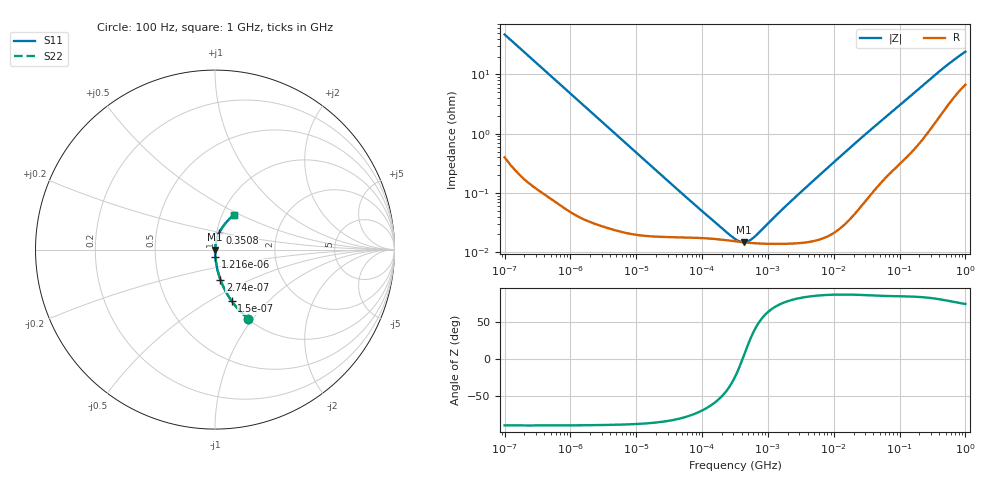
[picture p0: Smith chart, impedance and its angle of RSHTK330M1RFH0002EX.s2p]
! RSHTK330M1RFH0002EX  S-PARAMETER MODEL  (General Type)
! Model Generated by ELNA Corporation (http://www.ty-top.com)
! Version 1.0
! ELNA Control No. 201203
! Copyright (c) 2020 ELNA CO.,LTD. All Rights Reserved.
! Products Name : CONDUCTIVE POLYMER HYBRID ALUMINUM ELECTROLYTIC CAPACITORS
! Characteristics :
!  Capacitance  :  33uF  ,  Rated voltage  :  80V
!  Operating Temp. Range  :  -55 to +125 degC  ,  Endurance  :  4000hr at 125 degC
!  Dimension D  :  10mm  ,  Dimension L  :  10mm
! Frequency Range : 100Hz - 1GHz
! External Node Assignments :
!  1  o---| |---o  2
# MHz S RI R 50
!Freq[MHz].  S11 Real  S11 Imag  S21 Real  S21 Imag  S12 Real  S12 Imag  S22 Real  S22 Imag
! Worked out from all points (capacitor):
!   401 points, 100 Hz to 1 GHz, reference 50 ohm
!   read as one part in series: C = 33.6 uF near 108 Hz
!   lowest |Z| = 14.8 mohm at 436.5 kHz (marker M1)
!   series resonance near 412.7 kHz, so ESL is about 4.4 nH
!   S11 on the Smith chart (normalised r, x): 100 Hz: 1.01, -0.95; 150 Hz: 1.00, -0.63; 274 Hz: 1.00, -0.35; 1.216 kHz: 1.00, -0.08; 350.8 MHz: 1.03, +0.20; 1 GHz: 1.13, +0.47
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0.0001  0.1853 -0.3843  0.8147 0.3843  0.8147 0.3843  0.1853 -0.3843
0.00015  0.0928 -0.2866  0.9072 0.2866  0.9072 0.2866  0.0928 -0.2866
0.000274  0.0303 -0.1677  0.9697 0.1677  0.9697 0.1677  0.0303 -0.1677
0.000543  0.00834 -0.0867  0.9917 0.0867  0.9917 0.0867  0.00834 -0.0867
0.001216  0.00195 -0.0391  0.998 0.0391  0.998 0.0391  0.00195 -0.0391
0.001488  0.0014 -0.032  0.9986 0.032  0.9986 0.032  0.0014 -0.032
0.004241  0.000372 -0.0113  0.9996 0.0113  0.9996 0.0113  0.000372 -0.0113
0.022131  0.000187 -0.00217  0.9998 0.00217  0.9998 0.00217  0.000187 -0.00217
0.094406  0.000174 -0.000493  0.9998 0.000493  0.9998 0.000493  0.000174 -0.000493
0.316228  0.000153 -6.91e-05  0.9998 6.91e-05  0.9998 6.91e-05  0.000153 -6.91e-05
0.371535  0.00015 -2.73e-05  0.9999 2.73e-05  0.9999 2.73e-05  0.00015 -2.73e-05
0.436516  0.000147 1.48e-05  0.9999 -1.48e-05  0.9999 -1.48e-05  0.000147 1.48e-05
0.533949  0.000144 6.91e-05  0.9999 -6.91e-05  0.9999 -6.91e-05  0.000144 6.91e-05
0.653131  0.000142 0.000127  0.9999 -0.000127  0.9999 -0.000127  0.000142 0.000127
1.650061  0.000139 0.00051  0.9999 -0.00051  0.9999 -0.00051  0.000139 0.00051
4.704354  0.000155 0.00154  0.9998 -0.00154  0.9998 -0.00154  0.000155 0.00154
22.64644  0.000547 0.00737  0.9995 -0.00737  0.9995 -0.00737  0.000547 0.00737
69.9842  0.00255 0.0214  0.9975 -0.0214  0.9975 -0.0214  0.00255 0.0214
169.8244  0.00796 0.049  0.992 -0.049  0.992 -0.049  0.00796 0.049
350.7519  0.0244 0.0944  0.9756 -0.0944  0.9756 -0.0944  0.0244 0.0944
641.9482  0.0612 0.1501  0.9388 -0.1501  0.9388 -0.1501  0.0612 0.1501
1000  0.1057 0.1952  0.8943 -0.1952  0.8943 -0.1952  0.1057 0.1952
